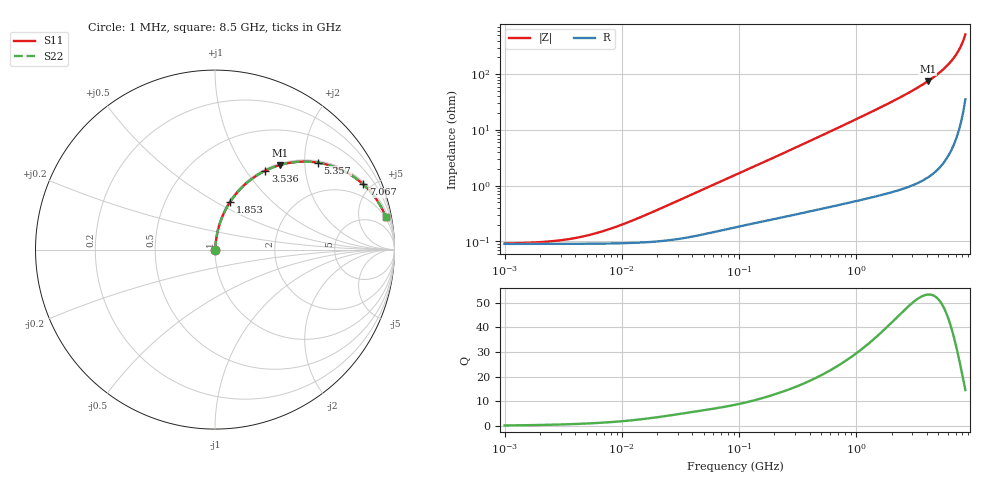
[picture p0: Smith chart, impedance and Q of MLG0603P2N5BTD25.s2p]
! S-Parameter Data Generated by TDK Corporation
! Copyright(C) 2025 TDK Corporation.
! All Rights Reserved.
! TDK P/N: MLG0603P2N5BTD25 (SMD / SMT Inductor (Coil))
! Property: L=2.5nH at 500MHz
! Size(LxWxT): 0.6x0.3x0.3mm
! Model Type: s2p (Touchstone File Format Version 1.0)
! Frequency: DC=Yes Start=1MHz Stop=8500MHz 198points Log-sweep
! Model Generated on Feb. 6, 2025
! Terms and conditions regarding TDK Simulation Models:
! 1)This simulation model is being provided solely for informational
!  purposes. Please refer to the specifications of the products in
!  terms of detailed characteristics of such products.
! 2)In no event shall TDK Corporation of any of its subsidiaries be
!  liable for any loss or damage arising, directly or indirectly,
!  from any information contained in this simulation model, including,
!  but not limited to loss or damages arising from any inaccuracies,
!  omissions or errors in connection with such information.
! 3)Any and all copyrights on this simulation model are owned by
!  TDK Corporation.  Duplication or redistribution of this simulation
!  model without prior written permission from TDK Corporation
!  is prohibited.
! 4)This simulation model is subject to any modification or change
!  without any prior notice.
! 5)Neither TDK Corporation nor any of its subsidiaries shall make any
!  warranty, express or implied, including but not limited to the
!  correctness, implied warranties of merchantability and fitness for
!  a particular purpose with respect to this simulation models.
! 6)The use of this simulation model shall be deemed to have consented
!  to the terms and conditions hereof.
! Port Assignments:
!  1 ---@@@--- 2
! Applicable Conditions:
!  Temperature = 25 degC
!  DC Bias Current = 0 A
!  Small Signal Operation
# Hz S MA R 50
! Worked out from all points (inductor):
!   197 points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, 1 MHz to 8.5 GHz, reference 50 ohm
!   read as one part in series: L = 2.8 nH near 16.71 MHz
!   highest Q = 53.4 at 4.061 GHz (marker M1), where L = 2.93 nH
!   S11 on the Smith chart (normalised r, x): 1 MHz: 1.00, +0.00; 1.853 GHz: 1.01, +0.59; 3.536 GHz: 1.02, +1.24; 5.357 GHz: 1.05, +2.32; 7.067 GHz: 1.14, +4.46; 8.5 GHz: 2, +10
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1000000  0.0009167 11.1  0.9991 -0.0  0.9991 -0.0  0.0009167 11.1
2403882  0.0009962 25.3  0.9991 -0.0  0.9991 -0.0  0.0009962 25.3
4587603  0.001216 41.9  0.9991 -0.0  0.9991 -0.0  0.001216 41.9
6337562  0.001444 50.9  0.9991 -0.1  0.9991 -0.1  0.001444 50.9
8755050  0.0018 59.2  0.9991 -0.1  0.9991 -0.1  0.0018 59.2
2.10461e7  0.00383 74.6  0.999 -0.2  0.999 -0.2  0.00383 74.6
9.219544e7  0.01539 82.5  0.9981 -0.9  0.9981 -0.9  0.01539 82.5
4.229561e8  0.06637 83.2  0.9943 -3.8  0.9943 -3.8  0.06637 83.2
9.270694e8  0.1427 79.8  0.9848 -8.2  0.9848 -8.2  0.1427 79.8
1.34121e9  0.2048 76.5  0.9729 -11.8  0.9729 -11.8  0.2048 76.5
1.852819e9  0.2809 72.3  0.9528 -16.3  0.9528 -16.3  0.2809 72.3
1.940355e9  0.2938 71.5  0.9488 -17.1  0.9488 -17.1  0.2938 71.5
2.680511e9  0.4018 65.1  0.9074 -23.7  0.9074 -23.7  0.4018 65.1
3.535948e9  0.5224 57.4  0.8428 -31.5  0.8428 -31.5  0.5224 57.4
4.061159e9  0.593 52.6  0.7941 -36.4  0.7941 -36.4  0.593 52.6
4.664383e9  0.6697 46.9  0.73 -42.0  0.73 -42.0  0.6697 46.9
5.357206e9  0.7503 40.2  0.6461 -48.6  0.6461 -48.6  0.7503 40.2
6.152938e9  0.8302 32.6  0.5385 -56.1  0.5385 -56.1  0.8302 32.6
7.066863e9  0.9023 23.8  0.4045 -64.4  0.4045 -64.4  0.9023 23.8
7.750377e9  0.9412 17.5  0.3008 -70.1  0.3008 -70.1  0.9412 17.5
8.116539e9  0.9569 14.2  0.2453 -72.9  0.2453 -72.9  0.9569 14.2
8.5e9  0.9694 10.8  0.1878 -75.3  0.1878 -75.3  0.9694 10.8
